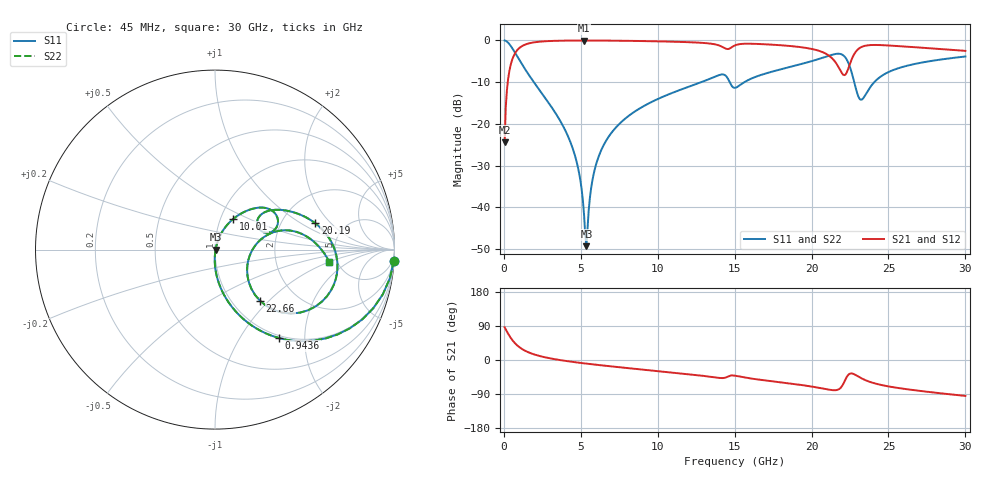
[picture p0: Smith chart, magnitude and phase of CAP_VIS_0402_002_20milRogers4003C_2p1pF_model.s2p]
! S-parameter model data by Modelithics Inc.  support@modelithics.com  813-866-6335  Tampa FL USA
! S-Parameter data specifications:
! Substrate: 20-mil Rogers 4003C, substrate thickness, H=0.508mm, Dielectric constant, Er=3.75
! PCB Mounting Pad Footprint: Pad width, PadW=0.50mm , Pad length, PadL=0.50mm , Pad gap, PadG (edge-to-edge)=0.40mm , Reference planes=1.4mm apart
! Created Wed Nov 18 12:44:21 2015
# hz S ma R 50
! 2 Port Network Data from SP1.SP block
! freq  magS11  angS11  magS21  angS21  magS12  angS12  magS22  angS22
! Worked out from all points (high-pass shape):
!   401 points, 45 MHz to 30 GHz, reference 50 ohm
!   highest |S21| = -0.03 dB at 5.212 GHz (marker M1); lowest = -24.4 dB at 45 MHz (marker M2)
!   |S21| within 3 dB of the highest: 732.2 MHz to 20.85 GHz (20.11 GHz wide, 186 % of centre); 22.81 GHz to end of sweep
!   lowest |S11| = -49.3 dB at 5.362 GHz (marker M3), VSWR 1.01, Z = 50.3 + j0.0141 ohm
!   |S11| at or under -10 dB: 1.947 GHz to 12.83 GHz (10.88 GHz wide, 147 % of centre); 14.68 GHz to 15.63 GHz (953 MHz wide, 6.29 % of centre); 22.77 GHz to 24.08 GHz (1.301 GHz wide, 5.56 % of centre)
!   |S22| runs from -49.3 to 0.0 dB; largest |S21 - S12| = 0
!   S11 on the Smith chart (normalised r, x): 45 MHz: 1, -32; 943.6 MHz: 0.96, -1.50; 10.01 GHz: 1.15, +0.41; 20.19 GHz: 3.08, +1.36; 22.66 GHz: 1.33, -0.89; 30 GHz: 4.32, -1.03
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4.5e7  0.9982 -3.5  0.06011 86.5  0.06011 86.5  0.9982 -3.5
4.194375e8  0.8706 -30.2  0.4916 59.8  0.4916 59.8  0.8706 -30.2
9.4365e8  0.6085 -54.1  0.7924 35.8  0.7924 35.8  0.6085 -54.1
1.992075e9  0.3078 -75.3  0.9495 14.4  0.9495 14.4  0.3078 -75.3
4.014038e9  0.0819 -90.4  0.9936 -2.4  0.9936 -2.4  0.0819 -90.4
4.688025e9  0.03758 -91.4  0.996 -6.2  0.996 -6.2  0.03758 -91.4
5.062462e9  0.01597 -86.3  0.9965 -8.1  0.9965 -8.1  0.01597 -86.3
5.212238e9  0.008066 -74.6  0.9965 -8.8  0.9965 -8.8  0.008066 -74.6
5.362012e9  0.003442 2.3  0.9965 -9.6  0.9965 -9.6  0.003442 2.3
5.886225e9  0.02767 70.6  0.9959 -12.0  0.9959 -12.0  0.02767 70.6
6.560212e9  0.05926 71.3  0.9943 -15.0  0.9943 -15.0  0.05926 71.3
1.000504e10  0.1989 59.2  0.9744 -29.2  0.9744 -29.2  0.1989 59.2
1.007992e10  0.2018 58.9  0.9738 -29.5  0.9738 -29.5  0.2018 58.9
1.412385e10  0.3904 31.4  0.8492 -47.7  0.8492 -47.7  0.3904 31.4
1.50225e10  0.2703 28.0  0.8717 -41.4  0.8717 -41.4  0.2703 28.0
2.003996e10  0.5667 16.1  0.788 -70.3  0.788 -70.3  0.5667 16.1
2.018974e10  0.5774 14.7  0.7767 -71.3  0.7767 -71.3  0.5774 14.7
2.176238e10  0.6926 -13.8  0.4758 -77.4  0.4758 -77.4  0.6926 -13.8
2.266102e10  0.3805 -48.7  0.6247 -35.8  0.6247 -35.8  0.3805 -48.7
2.326012e10  0.1953 -11.4  0.8366 -48.6  0.8366 -48.6  0.1953 -11.4
2.505742e10  0.4225 14.7  0.8679 -70.1  0.8679 -70.1  0.4225 14.7
3e10  0.6417 -6.3  0.7491 -94.8  0.7491 -94.8  0.6417 -6.3
